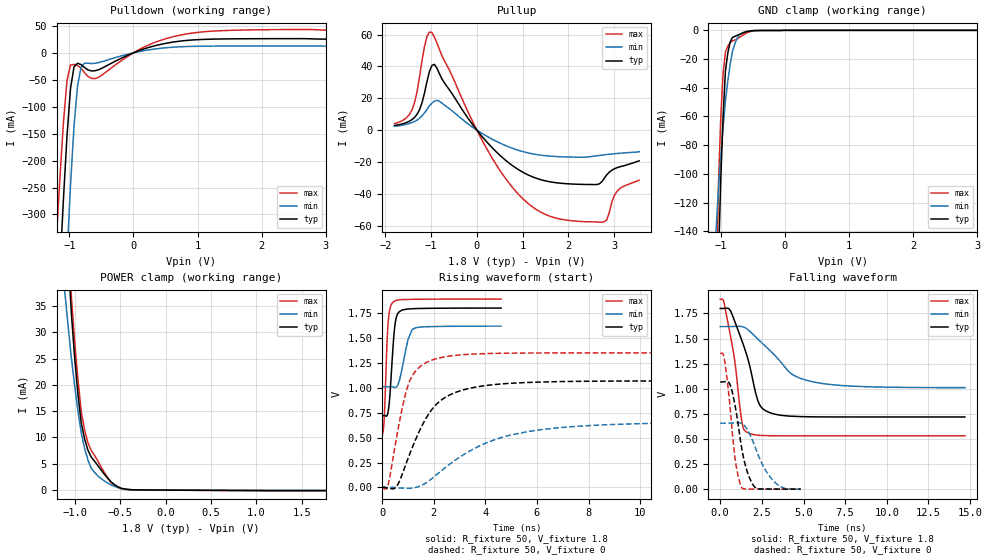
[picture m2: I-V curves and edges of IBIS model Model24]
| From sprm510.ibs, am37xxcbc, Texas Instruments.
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| Model based on original model for BQ18OMAPSMART1HYFBPBNOPM_SSBHH
|   Sub model NOPM_HS01L11_PU1_1P8
[model]   Model24
|[Input Load]   PU
|[Output Drive] SC01LB11
|Voltage   1.8V
|Mode   I/O
Model_type   I/O
Polarity   Non-Inverting
Enable   Active-Low
Vinl =  0.63
Vinh =  1.17
Cref =  15pF
Rref =  100.0000M
Vref =  0V
Vmeas =  0.9
C_comp   1.410688p   1.256095p   1.577871p
[Model Spec]
Vinl   0.63   0.567   0.6615
Vinh   1.17   1.053   1.2285
[Temperature Range]   25   125   -40
[Voltage Range]   1.8   1.62   1.89
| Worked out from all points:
|   slope of the pulldown table from 0 to 0.27 V, typ, clamps not added: 24.3 ohm
|   slope of the pullup table from 0 to 0.27 V, typ, clamps not added: 29.7 ohm
|   GND clamp passes 1 mA (typ) near -0.60 V on its own axis
|   POWER clamp passes 1 mA (typ) near -0.56 V on its own axis
|   rising waveform, R_fixture 50, V_fixture 1.8: 20-80 % time 174ps typ, 299ps min, 123ps max; typ from 0.72 V to 1.8 V
|   rising waveform, R_fixture 50, V_fixture 0: 20-80 % time 1.3ns typ, 2.85ns min, 686ps max; typ from 0.002 V to 1.07 V
|   falling waveform, R_fixture 50, V_fixture 1.8: 20-80 % time 1.1ns typ, 2.18ns min, 681ps max; typ from 1.8 V to 0.72 V
|   falling waveform, R_fixture 50, V_fixture 0: 20-80 % time 682ps typ, 1.11ns min, 499ps max; typ from 1.07 V to 0.001 V
[POWER_clamp]
-1.8V     362.5mA    191.4mA    412.8mA
-1.109V   56.76mA    37.74mA    60.51mA
-1.073V   44.67mA    31.25mA    47.93mA
-1.036V   33.52mA    25.07mA    36.72mA
-1V       25.06mA    19.75mA    28.2mA
-963.6mV  18.11mA    14.99mA    20.91mA
-927.3mV  12.67mA    10.8mA     14.87mA
-890.9mV  9.734mA    7.935mA    11.44mA
-818.2mV  6.293mA    4.153mA    7.536mA
-636.4mV  2.249mA    1.342mA    2.34mA
-418.2mV  128.7uA    129.3uA    104.4uA
1.764V    -96.73uA   -46.48uA   -163.5uA
[Pulldown]
-1.8V     -1.718A    -2.61A     -1.406A
-1.2V     -527.4mA   -844.5mA   -339.9mA
-1.145V   -396mA     -683.1mA   -229.1mA
-1.091V   -269mA     -526.7mA   -127.5mA
-1.036V   -153.6mA   -378.9mA   -51.17mA
-981.8mV  -66.33mA   -245.6mA   -22.67mA
-927.3mV  -26mA      -136.2mA   -21.54mA
-872.7mV  -19.34mA   -61.98mA   -23.69mA
-763.6mV  -27.2mA    -19.05mA   -36.72mA
-545.5mV  -31.39mA   -18.17mA   -45.46mA
872.7mV   23.46mA    11.88mA    35.92mA
3.545V    25.34mA    12.51mA    41.58mA
[Pullup]
-1.8V     2.903mA    2.423mA    4.112mA
-1.418V   6.595mA    4.711mA    12.64mA
-1.255V   12.69mA    7.42mA     33.24mA
-1.091V   30.4mA     13mA       58.69mA
-981.8mV  40.63mA    17.02mA    61.3mA
-818.2mV  35.38mA    18.12mA    50.59mA
272.7mV   -9.179mA   -4.728mA   -14.55mA
1.255V    -29.75mA   -15.09mA   -48.97mA
2.564V    -34.17mA   -16.31mA   -57.57mA
2.782V    -30.25mA   -15.5mA    -57.49mA
3.055V    -23.63mA   -14.68mA   -38.61mA
3.545V    -19.25mA   -13.56mA   -31.41mA
[GND_clamp]
-1.8V     -2.82A     -1.192A    -3.165A
-1.073V   -235.8mA   -138.4mA   -192.1mA
-1.036V   -159.6mA   -110.8mA   -107.6mA
-1V       -103.8mA   -87.86mA   -60.73mA
-963.6mV  -60.04mA   -67.29mA   -29.86mA
-927.3mV  -28.26mA   -49.09mA   -14.98mA
-890.9mV  -15.95mA   -35.49mA   -11.09mA
-854.5mV  -8.198mA   -24.09mA   -8.559mA
-818.2mV  -4.99mA    -14.87mA   -7.387mA
-709.1mV  -2.858mA   -3.093mA   -5.012mA
-527.3mV  -395.6uA   -260.4uA   -751.2uA
3.6V      0A         0A         0A
[Ramp]
dV/dt_f  0.6499156/1.098495n   0.366978/2.193507n   0.8166769/0.6836084n
dV/dt_r   0.649755/1.301947n   0.4004131/2.877975n   0.8202155/0.6872151n
R_load = 50
[Rising Waveform]
R_fixture = 50
V_fixture = 1.8
V_fixture_min = 1.62
V_fixture_max = 1.89
0s        720mV      1.011V     529.4mV
81ps      721.7mV    1.011V     710.8mV
180ps     718.8mV    1.011V     1.417V
234ps     768mV      1.011V     1.669V
297ps     928.1mV    1.012V     1.791V
387ps     1.288V     1.011V     1.849V
486ps     1.617V     1.003V     1.87V
567ps     1.724V     1.012V     1.879V
1.161ns   1.793V     1.584V     1.887V
4.608ns   1.799V     1.618V     1.89V
[Rising Waveform]
R_fixture = 50
V_fixture = 0
V_fixture_min = 0
V_fixture_max = 0
0s        1.569mV    1.041mV    -8.828mV
225ps     -8.247mV   908.7uV    25.48mV
585ps     21.65mV    -2.894mV   542.9mV
855ps     190mV      -7.114mV   887.8mV
1.08ns    345.2mV    -8.118mV   1.076V
1.629ns   662.2mV    35.07mV    1.242V
2.124ns   840.2mV    132mV      1.294V
3.996ns   1.022V     443mV      1.343V
6.192ns   1.058V     581.1mV    1.349V
19.59ns   1.069V     657.1mV    1.35V
[Falling Waveform]
R_fixture = 50
V_fixture = 1.8
V_fixture_min = 1.62
V_fixture_max = 1.89
0s        1.8V       1.62V      1.89V
198ps     1.8V       1.62V      1.876V
594ps     1.783V     1.62V      1.546V
1.323ns   1.47V      1.619V     655.2mV
1.62ns    1.321V     1.594V     566.9mV
2.376ns   837.7mV    1.477V     537.3mV
3.168ns   752.7mV    1.352V     533.3mV
4.293ns   727.6mV    1.148V     532.6mV
5.688ns   721.2mV    1.066V     532.6mV
14.69ns   720mV      1.012V     532.6mV
[Falling Waveform]
R_fixture = 50
V_fixture = 0
V_fixture_min = 0
V_fixture_max = 0
0s        1.069V     658.6mV    1.35V
270ps     1.071V     658.7mV    1.275V
648ps     1.015V     659.1mV    717.2mV
945ps     785.4mV    662.3mV    249.1mV
1.287ns   414.4mV    655.7mV    18.8mV
1.611ns   181.5mV    599.7mV    3.599mV
2.097ns   18.9mV     420.4mV    2.003mV
2.664ns   2.936mV    207.1mV    1.798mV
3.33ns    1.734mV    61.82mV    1.775mV
4.833ns   1.436mV    2.601mV    1.773mV
